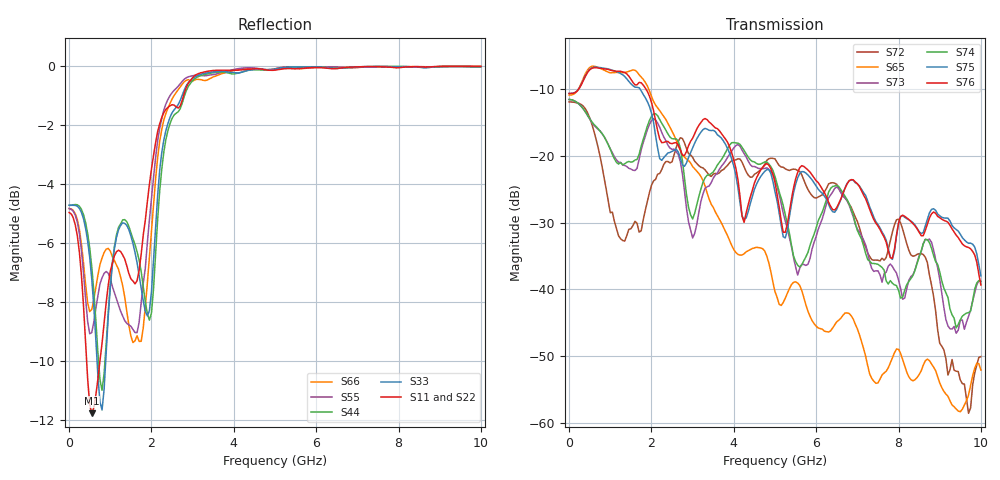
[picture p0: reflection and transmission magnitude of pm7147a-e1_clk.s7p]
# GHz S DB R 50
! S-Parameters data
! Freq  dbS11  angS11  dbS12  angS12  dbS13  angS13  dbS14  angS14
!  dbS15  angS15  dbS16  angS16  dbS17  angS17  dbS21  angS21
!  dbS22  angS22  dbS23  angS23  dbS24  angS24  dbS25  angS25
!  dbS26  angS26  dbS27  angS27  dbS31  angS31  dbS32  angS32
!  dbS33  angS33  dbS34  angS34  dbS35  angS35  dbS36  angS36
!  dbS37  angS37  dbS41  angS41  dbS42  angS42  dbS43  angS43
!  dbS44  angS44  dbS45  angS45  dbS46  angS46  dbS47  angS47
!  dbS51  angS51  dbS52  angS52  dbS53  angS53  dbS54  angS54
!  dbS55  angS55  dbS56  angS56  dbS57  angS57  dbS61  angS61
!  dbS62  angS62  dbS63  angS63  dbS64  angS64  dbS65  angS65
!  dbS66  angS66  dbS67  angS67  dbS71  angS71  dbS72  angS72
!  dbS73  angS73  dbS74  angS74  dbS75  angS75  dbS76  angS76
!  dbS77  angS77
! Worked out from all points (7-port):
!   279 points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, 1 Hz to 10 GHz, reference 50 ohm
!   strongest paths, dB at 1 Hz, 7.943 MHz, 3.05 GHz, 6.55 GHz, 10 GHz:
!     S76: -10.6, -10.6, -16.6, -27.1, -39.4
!     S75: -10.6, -10.6, -18.1, -27.3, -38.0
!     S74: -11.5, -11.5, -28.6, -24.6, -38.8
!     S73: -11.5, -11.5, -31.6, -25.0, -38.8
!     S65: -10.9, -10.9, -21.9, -44.6, -52.1
!     S72: -11.9, -11.9, -20.8, -24.8, -50.1
!   lowest |S11| = -11.8 dB at 550 MHz (marker M1), VSWR 1.70, Z = 29.5 + j1.15 ohm
!   |S11| at or under -10 dB: 425.6 MHz to 748.2 MHz (322.6 MHz wide, 55 % of centre)
